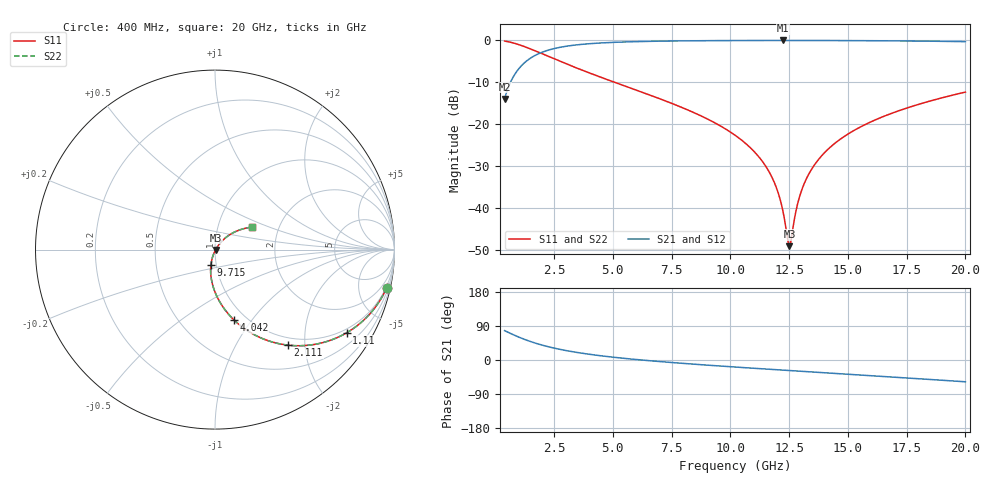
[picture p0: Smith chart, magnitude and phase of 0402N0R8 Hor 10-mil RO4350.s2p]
# GHz S MA R 50
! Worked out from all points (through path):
!   1960 points, 400 MHz to 20 GHz, reference 50 ohm
!   highest |S21| = -0.03 dB at 12.25 GHz (marker M1); lowest = -14.0 dB at 400 MHz (marker M2)
!   lowest |S11| = -49.1 dB at 12.52 GHz (marker M3), VSWR 1.01, Z = 50.3 - j0.164 ohm
!   |S11| at or under -10 dB: 5.074 GHz to end of sweep
!   |S22| runs from -49.1 to -0.2 dB; largest |S21 - S12| = 0
!   S11 on the Smith chart (normalised r, x): 400 MHz: 0.86, -9.06; 1.11 GHz: 0.86, -3.25; 2.111 GHz: 0.87, -1.68; 4.042 GHz: 0.88, -0.82; 9.715 GHz: 0.94, -0.17; 20 GHz: 1.46, +0.39
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0.4  0.9796 -12.5  0.2007 77.5  0.2007 77.5  0.9796 -12.5
0.7401736  0.9347 -22.5  0.355 67.5  0.355 67.5  0.9347 -22.5
1.110362  0.8679 -32.3  0.4961 57.7  0.4961 57.7  0.8679 -32.3
2.110873  0.6706 -52.6  0.7407 37.4  0.7407 37.4  0.6706 -52.6
3.671669  0.4437 -71.7  0.8945 18.1  0.8945 18.1  0.4437 -71.7
4.041858  0.4047 -75.0  0.9126 14.8  0.9126 14.8  0.4047 -75.0
6.943338  0.2038 -93.2  0.9764 -3.8  0.9764 -3.8  0.2038 -93.2
9.714752  0.09063 -104.7  0.9926 -16.5  0.9926 -16.5  0.09063 -104.7
10.205  0.07382 -106.2  0.9938 -18.6  0.9938 -18.6  0.07382 -106.2
10.9754  0.04846 -108.0  0.9952 -21.7  0.9952 -21.7  0.04846 -108.0
11.54569  0.03035 -107.7  0.9957 -24.0  0.9957 -24.0  0.03035 -107.7
11.9559  0.01765 -104.5  0.9959 -25.6  0.9959 -25.6  0.01765 -104.5
12.24604  0.009011 -94.2  0.996 -26.8  0.996 -26.8  0.009011 -94.2
12.43614  0.004275 -62.5  0.996 -27.5  0.996 -27.5  0.004275 -62.5
12.51618  0.003519 -27.7  0.996 -27.8  0.996 -27.8  0.003519 -27.7
12.58622  0.004144 3.4  0.9959 -28.1  0.9959 -28.1  0.004144 3.4
12.78632  0.009042 37.8  0.9958 -28.9  0.9958 -28.9  0.009042 37.8
12.95641  0.01399 45.5  0.9957 -29.6  0.9957 -29.6  0.01399 45.5
13.46667  0.02933 51.1  0.9953 -31.5  0.9953 -31.5  0.02933 51.1
14.7073  0.06715 50.2  0.9931 -36.4  0.9931 -36.4  0.06715 50.2
16.73834  0.1308 43.7  0.9862 -44.3  0.9862 -44.3  0.1308 43.7
20  0.2416 31.2  0.9641 -57.5  0.9641 -57.5  0.2416 31.2
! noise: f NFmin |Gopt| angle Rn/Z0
0.4  0.001416  0.8453  5.958  0.001939
2.571  0.00504  0.6824  8.988  0.003055
4.752  0.00801  0.6368  12.89  0.004106
6.933  0.01073  0.6109  17.08  0.005008
9.104  0.01333  0.5949  21.29  0.005851
11.29  0.01593  0.5854  25.49  0.006696
13.47  0.01858  0.5809  29.62  0.007578
15.64  0.02131  0.5806  33.65  0.008529
17.82  0.02422  0.5841  37.61  0.009592
20  0.02733  0.591  41.48  0.01081
